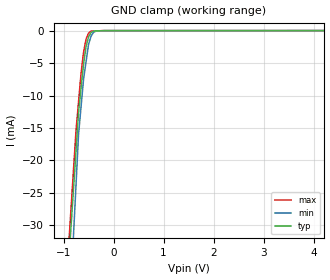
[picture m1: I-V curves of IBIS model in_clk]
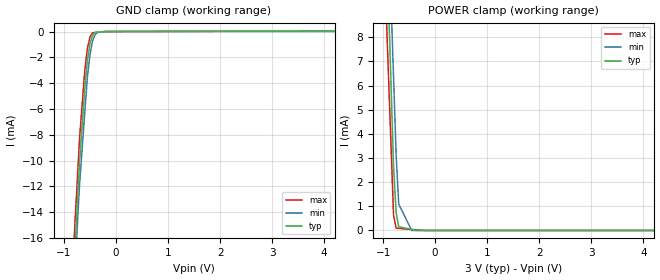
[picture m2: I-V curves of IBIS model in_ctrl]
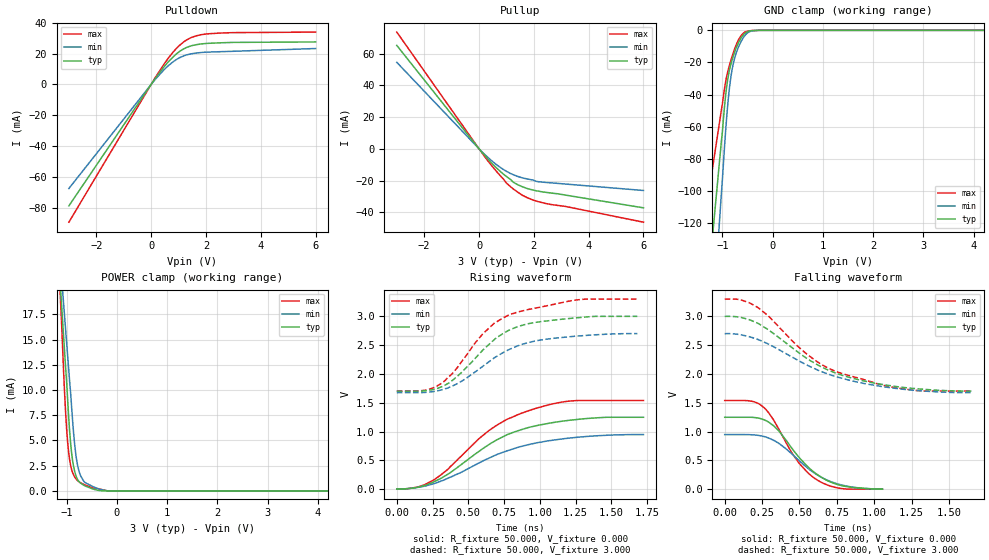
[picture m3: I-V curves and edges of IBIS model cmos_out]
| Teraspeed (R) Labs.
| http://www.teraspeed.com
[IBIS Ver]   3.2
[Comment Char] |_char
[File Name]   ads1672.ibs
[File Rev]   3.0
[Source]
| This model file was created by Teraspeed Consulting Group LLC
| (http://www.teraspeed.com/).
[Date]   06-03-2010
[Notes]   Quality Check of this IBIS model: Model Passes IBIS Check
   Model parses into ICX IS. Simulation done with Hyperlynx.
   Ver 1.0 09-18-2008
   1. MIN TYP MAX information is based on Temperature and Voltage
   characteristics only.
   Ver 2.0 06-03-10
   2. LVDS buffer updated
[Disclaimer]
| This product is designed as an aid for customers of Texas Instruments.
| No warranties, either expressed or implied, with respect to this third
| party software (if any) or with respect to its fitness for any
| particular purpose is claimed by Texas Instruments or the author. The
| software (if any) is provided solely on an "as is" basis. The entire
| risk as to its quality and performance is with the customer
[Copyright]
| (C) Copyright 2008 Texas Instruments Incorporated. All rights reserved.
| All other rights are reserved.
[Component]   ADS1672
[Manufacturer] TI
[Package]
| variable   typ   min   max
R_pkg  1.685E-02  1.414E-02  1.967E-02
L_pkg  1.643E-09  1.379E-09  1.918E-09
C_pkg  3.888E-13  3.264E-13  4.540E-13
[Pin] signal_name  model_name  R_pin  L_pin C_pin
1   AVDD   POWER   1.967E-02 1.918E-09 4.540E-13
2   AGND   GND   1.885E-02 1.838E-09 4.350E-13
3   AGND   GND   1.803E-02 1.758E-09 4.160E-13
4   AINN   term   1.721E-02 1.678E-09 3.970E-13
5   AINP   term   1.640E-02 1.599E-09 3.785E-13
6   AGND   GND   1.562E-02 1.523E-09 3.605E-13
7   AVDD   POWER   1.487E-02 1.449E-09 3.431E-13
8   RBIAS   term   1.414E-02 1.379E-09 3.264E-13
9   AGND   GND   1.414E-02 1.379E-09 3.264E-13
10  AGND   GND   1.487E-02 1.449E-09 3.431E-13
11  AVDD   POWER   1.562E-02 1.523E-09 3.605E-13
12  AVDD   POWER   1.640E-02 1.599E-09 3.785E-13
13  VCM   term   1.721E-02 1.678E-09 3.970E-13
14  DGND   GND   1.803E-02 1.758E-09 4.160E-13
15  DGND   GND   1.885E-02 1.838E-09 4.350E-13
16  DGND   GND   1.967E-02 1.918E-09 4.540E-13
17  DGND   GND   1.967E-02 1.918E-09 4.540E-13
18  DGND   GND   1.885E-02 1.838E-09 4.350E-13
19  DGND   GND   1.803E-02 1.758E-09 4.160E-13
20  DGND   GND   1.721E-02 1.678E-09 3.970E-13
21  RSV2   term   1.640E-02 1.599E-09 3.785E-13
22  RSV1   term   1.562E-02 1.523E-09 3.605E-13
23  DVDD   POWER   1.487E-02 1.449E-09 3.431E-13
24  DVDD   POWER   1.414E-02 1.379E-09 3.264E-13
25  DGND   GND   1.414E-02 1.379E-09 3.264E-13
26  DGND   GND   1.487E-02 1.449E-09 3.431E-13
27  DVDD   POWER   1.562E-02 1.523E-09 3.605E-13
28  *PDWN   in_ctrl   1.640E-02 1.599E-09 3.785E-13
29  SCLK_SEL  in_ctrl   1.721E-02 1.678E-09 3.970E-13
30  *LVDS   in_ctrl   1.803E-02 1.758E-09 4.160E-13
31  DGND   GND   1.885E-02 1.838E-09 4.350E-13
32  LL_CONFIG in_ctrl   1.967E-02 1.918E-09 4.540E-13
33  FPATH   in_ctrl   1.967E-02 1.918E-09 4.540E-13
34  DVDD   POWER   1.885E-02 1.838E-09 4.350E-13
35  DRATE[1]  in_ctrl   1.803E-02 1.758E-09 4.160E-13
36  DRATE[0]  in_ctrl   1.721E-02 1.678E-09 3.970E-13
37  START   in_ctrl   1.640E-02 1.599E-09 3.785E-13
38  *CS   in_ctrl   1.562E-02 1.523E-09 3.605E-13
39  OTRD   cmos_out  1.487E-02 1.449E-09 3.431E-13
40  RSV3   NC   1.414E-02 1.379E-09 3.264E-13
41  *SCLK   output   1.414E-02 1.379E-09 3.264E-13
42  SCLK   output   1.487E-02 1.449E-09 3.431E-13
43  *DOUT   output   1.562E-02 1.523E-09 3.605E-13
44  DOUT   output   1.640E-02 1.599E-09 3.785E-13
45  *DRDY   output   1.721E-02 1.678E-09 3.970E-13
46  DRDY   output   1.803E-02 1.758E-09 4.160E-13
47  DGND   GND   1.885E-02 1.838E-09 4.350E-13
48  DVDD   POWER   1.967E-02 1.918E-09 4.540E-13
49  DVDD   POWER   1.967E-02 1.918E-09 4.540E-13
50  DGND   GND   1.885E-02 1.838E-09 4.350E-13
51  DGND   GND   1.803E-02 1.758E-09 4.160E-13
52  DVDD   POWER   1.721E-02 1.678E-09 3.970E-13
53  AVDD   POWER   1.640E-02 1.599E-09 3.785E-13
54  AGND   GND   1.562E-02 1.523E-09 3.605E-13
55  CLK   in_clk   1.487E-02 1.449E-09 3.431E-13
56  AGND   GND   1.414E-02 1.379E-09 3.264E-13
57  AGND   GND   1.414E-02 1.379E-09 3.264E-13
58  AVDD   POWER   1.487E-02 1.449E-09 3.431E-13
59  CAP1   term   1.562E-02 1.523E-09 3.605E-13
60  VREFN   GND   1.640E-02 1.599E-09 3.785E-13
61  VREFN   GND   1.721E-02 1.678E-09 3.970E-13
62  CAP2   term   1.803E-02 1.758E-09 4.160E-13
63  VREFP   POWER   1.885E-02 1.838E-09 4.350E-13
64  VREFP   POWER   1.967E-02 1.918E-09 4.540E-13
[Diff Pin] inv_pin vdiff tdelay_typ tdelay_min tdelay_max
5   4   NA  NA  NA  NA
42  41  NA  NA  NA  NA
44  43  NA  NA  NA  NA
46  45  NA  NA  NA  NA
[Model Selector]  output
cmos_out  cmos mode output(*lvds=1)
lvds_out  lvds mode output(*lvds=0)
[Model] term
Model_type Terminator
C_comp   0  0  0
| variable   typ   min   max
[Voltage Range]   5.00000V  4.75000V  5.25000V
[POWER Clamp Reference]  5.00000V  4.75000V  5.25000V
[GND Clamp Reference]   0.00000V  0.00000V  0.00000V
[Temperature Range]   25   85   -40
| Models and submodels in the file (5): in_clk (Input), in_ctrl (Input), cmos_out (Output), lvds_out (Output), term (Terminator)
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[Model] in_clk
Model_type Input
Vinl = 900.000mV
Vinh = 2.10000V
C_comp 1.290pF 1.290pF 1.290pF
| variable typ   min   max
[Voltage Range] 3.00000V 2.70000V 3.30000V
[POWER Clamp Reference] 3.00000V 2.70000V 3.30000V
[GND Clamp Reference] 0.00000V 0.00000V 0.00000V
[Temperature Range]   25   85   -40
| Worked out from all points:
|   GND clamp passes 1 mA (typ) near -0.50 V on its own axis
[GND Clamp]
-3V       -281.8mA   -369.5mA   -286.2mA
-750mV    -18.45mA   -23.69mA   -15.34mA
-700mV    -12.6mA    -16mA      -10.97mA
-650mV    -8.861mA   -11.75mA   -6.601mA
-600mV    -5.124mA   -7.494mA   -3.35mA
-550mV    -2.495mA   -4.812mA   -1.316mA
-500mV    -966.6uA   -2.129mA   -388.7uA
-450mV    -284.6uA   -840.9uA   -86.6uA
-400mV    -67.21uA   -264uA     -67.67uA
-350mV    -51.36uA   -70.85uA   -48.74uA
-175mV    -3.78uA    -4.485uA   -1.369uA
6V        5.589uA    5.808uA    3.751uA
[POWER Clamp]
-3V       0A         0A         0A
6V        0A         0A         0A
[Model] in_ctrl
Model_type Input
Vinl = 900.000mV
Vinh = 2.10000V
C_comp 1.430pF 1.430pF 1.430pF
| variable typ   min   max
[Voltage Range] 3.00000V 2.70000V 3.30000V
[POWER Clamp Reference] 3.00000V 2.70000V 3.30000V
[GND Clamp Reference] 0.00000V 0.00000V 0.00000V
[Temperature Range]   25   85   -40
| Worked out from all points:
|   GND clamp passes 1 mA (typ) near -0.50 V on its own axis
|   POWER clamp passes 1 mA (typ) near -0.76 V on its own axis
[GND Clamp]
-3V       -183mA     -184.7mA   -179.2mA
-700mV    -10.17mA   -11.86mA   -8.283mA
-600mV    -4.431mA   -6.327mA   -3.042mA
-550mV    -2.286mA   -3.562mA   -1.318mA
-500mV    -938.6uA   -1.813mA   -425.2uA
-450mV    -289.7uA   -733.7uA   -101.1uA
-400mV    -70.38uA   -231.8uA   -79uA
-350mV    -53.44uA   -61.49uA   -56.87uA
-225mV    -11.08uA   -20.62uA   -1.535uA
-200mV    -2.614uA   -12.44uA   -1.314uA
-175mV    -2.301uA   -4.267uA   -1.093uA
6V        74.87uA    9.554uA    53.52uA
[POWER Clamp]
-3V       157.8mA    148.7mA    141.2mA
-1.05V    20.28mA    22.54mA    15.53mA
-800mV    2.647mA    6.365mA    643.6uA
-750mV    736.9uA    3.131mA    95.44uA
-700mV    153.2uA    1.089mA    86.35uA
-450mV    43.76uA    38.81pA    40.9uA
-350mV    0A         0A         22.72uA
6V        0A         0A         0A
[Model]   cmos_out
Model_type Output
Vref=0.000E+00
Rref=1.000E+06
Cref=0.000E+00
Vmeas=1.500E+00
C_comp   1.220E-12   1.220E-12   1.220E-12
[Voltage Range]   3.000E+00   2.700E+00   3.300E+00
[POWER Clamp Reference]   3.000E+00   2.700E+00   3.300E+00
[GND Clamp Reference]   0.000E+00   0.000E+00   0.000E+00
[Pullup Reference]   3.000E+00   2.700E+00   3.300E+00
[Pulldown Reference]   0.000E+00   0.000E+00   0.000E+00
[Temperature Range]   25   85   -40
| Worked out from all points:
|   slope of the pulldown table from 0 to 0.45 V, typ, clamps not added: 41.2 ohm
|   slope of the pullup table from 0 to 0.45 V, typ, clamps not added: 51 ohm
|   GND clamp passes 1 mA (typ) near -0.51 V on its own axis
|   POWER clamp passes 1 mA (typ) near -0.77 V on its own axis
|   rising waveform, R_fixture 50.000, V_fixture 0.000: 20-80 % time 478ps typ, 540ps min, 450ps max; typ from 0 V to 1.25 V
|   falling waveform, R_fixture 50.000, V_fixture 0.000: 20-80 % time 255ps typ, 278ps min, 228ps max; typ from 1.25 V to 0 V
|   rising waveform, R_fixture 50.000, V_fixture 3.000: 20-80 % time 346ps typ, 396ps min, 355ps max; typ from 1.7 V to 3 V
|   falling waveform, R_fixture 50.000, V_fixture 3.000: 20-80 % time 500ps typ, 539ps min, 466ps max; typ from 3 V to 1.7 V
[GND Clamp]
-3V       -732.5mA   -1.011A    -457.5mA
-1.02V    -68.96mA   -101.5mA   -49.48mA
-940mV    -41.7mA    -64.41mA   -32.72mA
-900mV    -31.74mA   -48.47mA   -26.58mA
-860mV    -24.8mA    -35.95mA   -21.78mA
-820mV    -19.71mA   -26.78mA   -17.56mA
-780mV    -15.63mA   -20.27mA   -13.68mA
-720mV    -10.51mA   -13.58mA   -8.589mA
-640mV    -5.387mA   -7.697mA   -3.855mA
-540mV    -1.541mA   -2.736mA   -904.2uA
-280mV    0A         0A         0A
6V        0A         0A         0A
[Power Clamp]
-3V       165.6mA    142.9mA    228.4mA
-1.12V    20.03mA    22.45mA    18.8mA
-1.1V     18.48mA    21.17mA    16.72mA
-1.06V    15.38mA    18.6mA     11.93mA
-1.02V    12.29mA    16.04mA    7.842mA
-980mV    9.147mA    13.48mA    4.886mA
-940mV    5.972mA    10.92mA    3.099mA
-880mV    3mA        6.947mA    1.825mA
-800mV    1.324mA    3.058mA    1.12mA
-620mV    466uA      790.6uA    567.5uA
-180mV    0A         0A         0A
6V        0A         0A         0A
[Pullup]
-3V       65.09mA    54.44mA    73.48mA
180mV     -3.633mA   -3.142mA   -4.285mA
680mV     -12.72mA   -10.54mA   -15.09mA
1V        -17.45mA   -14.18mA   -21.54mA
1.26V     -21.11mA   -16.39mA   -25.43mA
1.74V     -24.9mA    -18.92mA   -30.63mA
2.18V     -26.71mA   -20.75mA   -33.37mA
6V        -37.17mA   -26.26mA   -46.21mA
[Pulldown]
-3V       -78.82mA   -67.55mA   -89.4mA
160mV     4.106mA    3.474mA    4.698mA
500mV     12.03mA    10.05mA    13.92mA
780mV     17.48mA    14.4mA     20.51mA
1V        20.92mA    17mA       24.8mA
1.18V     22.99mA    18.48mA    27.49mA
1.44V     24.96mA    19.81mA    30.26mA
1.62V     25.72mA    20.34mA    31.45mA
2.1V      26.71mA    21.04mA    32.91mA
2.98V     27.3mA     21.53mA    33.65mA
6V        27.6mA     23.33mA    34mA
[Rising Waveform]
R_fixture = 50.000
V_fixture = 0.000
V_fixture_min = 0.000
V_fixture_max = 0.000
|  time   V(typ)   V(min)   V(max)
0s        0V         0V         0V
157.5ps   39.12mV    35.27mV    45.19mV
262.5ps   130.7mV    97.67mV    165.6mV
357.5ps   259.3mV    190.7mV    344.7mV
645ps     774.7mV    538.7mV    1.019V
770ps     944mV      664.6mV    1.212V
877.5ps   1.038V     746.5mV    1.323V
1.065ns   1.144V     841.3mV    1.467V
1.21ns    1.197V     887.9mV    1.53V
1.725ns   1.248V     948mV      1.539V
[Falling Waveform]
R_fixture = 50.000
V_fixture = 0.000
V_fixture_min = 0.000
V_fixture_max = 0.000
|  time   V(typ)   V(min)   V(max)
0s        1.248V     948mV      1.539V
182.5ps   1.247V     944.1mV    1.526V
265ps     1.202V     912.5mV    1.41V
357.5ps   1.024V     803.2mV    1.063V
442.5ps   733.7mV    626.7mV    659.1mV
500ps     543.3mV    490.1mV    443.1mV
567.5ps   360.6mV    339.9mV    258.3mV
637.5ps   222mV      219.1mV    130.5mV
787.5ps   57.84mV    68.99mV    9.496mV
1.055ns   0V         0V         0V
[Rising Waveform]
R_fixture = 50.000
V_fixture = 3.000
V_fixture_min = 2.700
V_fixture_max = 3.300
|  time   V(typ)   V(min)   V(max)
0s        1.702V     1.676V     1.703V
202.5ps   1.709V     1.68V      1.72V
315ps     1.779V     1.725V     1.839V
432.5ps   1.98V      1.843V     2.14V
602.5ps   2.416V     2.135V     2.699V
682.5ps   2.597V     2.28V      2.882V
802.5ps   2.78V      2.443V     3.041V
987.5ps   2.901V     2.582V     3.152V
1.255ns   2.974V     2.656V     3.284V
1.682ns   3V         2.7V       3.3V
[Falling Waveform]
R_fixture = 50.000
V_fixture = 3.000
V_fixture_min = 2.700
V_fixture_max = 3.300
|  time   V(typ)   V(min)   V(max)
0s        3V         2.7V       3.3V
110ps     2.981V     2.68V      3.284V
217.5ps   2.884V     2.603V     3.159V
290ps     2.77V      2.522V     3.011V
547.5ps   2.273V     2.158V     2.349V
645ps     2.126V     2.043V     2.168V
747.5ps   2.011V     1.951V     2.04V
1.165ns   1.775V     1.743V     1.752V
1.325ns   1.735V     1.705V     1.705V
1.65ns    1.702V     1.676V     1.703V
[Ramp]
dV/dt_r   7.4912E-01/4.7767E-10   5.6820E-01/5.3971E-10   9.2374E-01/4.4764E-10
dV/dt_f   7.7859E-01/4.9910E-10   6.1419E-01/5.3846E-10   9.5808E-01/4.6493E-10
R_load = 50
